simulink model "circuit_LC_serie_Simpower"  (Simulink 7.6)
settings: Solver=ode15s  StartTime=0.0  StopTime=0.0035  RelTol=1e-3
InitFcn:
  | clc, close all,clear all
  | R=10;
  | C=1e-6;
  | L=1e-3;
StopFcn:
  | close all
  | load tension_Vc.mat
  | plot(x(1,:),x(2,:))
  | hold on
  | plot(x(1,:),x(3,:))
  | %axis([0 0.04 -20 1020])
  | grid
  | title('Tension aux bornes du circuit LC série et créneau d''entrée')
  | xlabel('temps')
libraries: powerlib x9

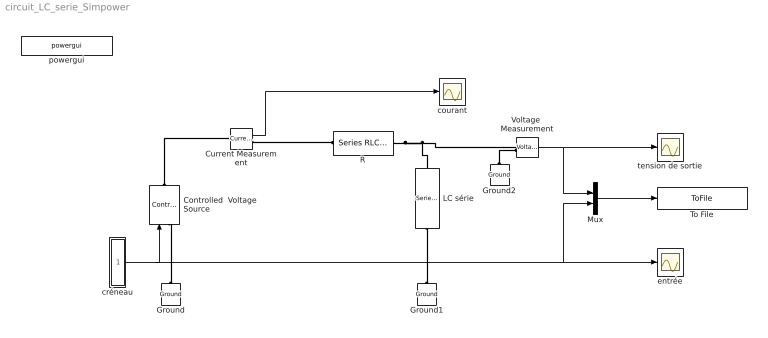
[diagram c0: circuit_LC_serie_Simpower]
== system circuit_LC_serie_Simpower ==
  Controlled  Voltage Source : powerlib/Electrical Sources/Controlled Voltage Source  DialogController=POWERSYS.PowerSysDialog  SystemSampleTime=-1  Initialize=on  Source_Type=AC  Amplitude=0  Phase=0  Frequency=0  Measurements=None
  Current Measurement : powerlib/Measurements/Current Measurement  DialogController=POWERSYS.PowerSysDialog  SystemSampleTime=-1  PhasorSimulation=off  OutputType=Complex  PSBequivalent=0
  Ground : powerlib/Elements/Ground  DialogController=POWERSYS.PowerSysDialog  PhysicalDomain=powersysdomain  SubClassName=unknown  LeftPortType=p1  RightPortType=p1  LConnTagsString=a
  Ground1 : powerlib/Elements/Ground  DialogController=POWERSYS.PowerSysDialog  PhysicalDomain=powersysdomain  SubClassName=unknown  LeftPortType=p1  RightPortType=p1  LConnTagsString=a
  Ground2 : powerlib/Elements/Ground  DialogController=POWERSYS.PowerSysDialog  PhysicalDomain=powersysdomain  SubClassName=unknown  LeftPortType=p1  RightPortType=p1  LConnTagsString=a
  LC série : powerlib/Elements/Series RLC Branch  DialogController=POWERSYS.PowerSysDialog  PhysicalDomain=powersysdomain  SubClassName=unknown  LeftPortType=p1  RightPortType=p1  LConnTagsString=__new0  RConnTagsString=__new0  BranchType=LC  Resistance=10  Inductance=L  SetiL0=off  InitialCurrent=0  Capacitance=C  Setx0=off  InitialVoltage=0  Measurements=None
  Mux : Mux  Inputs=2
  R : powerlib/Elements/Series RLC Branch  DialogController=POWERSYS.PowerSysDialog  PhysicalDomain=powersysdomain  SubClassName=unknown  LeftPortType=p1  RightPortType=p1  LConnTagsString=__new0  RConnTagsString=__new0  BranchType=R  Resistance=R  Inductance=1e-3  SetiL0=off  InitialCurrent=0  Capacitance=1e-6  Setx0=off  InitialVoltage=0  Measurements=None
  To File : ToFile  Filename=tension_Vc.mat  MatrixName=x
  Voltage  Measurement : powerlib/Measurements/Voltage Measurement  DialogController=POWERSYS.PowerSysDialog  SystemSampleTime=-1  PhasorSimulation=off  OutputType=Complex  PSBequivalent=0
  courant : Scope
  créneau : Subsystem
  entrée : Scope
  powergui : powerlib/powergui  Priority=1  SystemSampleTime=-1  SimulationMode=Continuous  SampleTime=50e-6  frequency=60  SPID=off  DisableSnubberDevices=off  DisableRonSwitches=off  DisableVfSwitches=off  SwTol=0  Interpol=off  frequencyindice=0  echomessages=off  HookPort=off  DisplayEquations=off  FunctionMessages=off  EnableUseOfTLC=off  x0status=blocks  RestoreLinks=warning  ResistiveCurrentMeasurement=off  Ylog=off  Xlog=on  ShowGrid=off  save=off  variable=ZData  ZoomFFT=off  StartTime=0.0  cycles=1  DisplayStyle=1  fundamental=60  FreqAxis=off  MaxFrequency=1000  frequencyindicesteady=1  display=off  methode=off
  tension de sortie : Scope
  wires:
  Current Measurement/1 -> courant/1
  Voltage  Measurement/1 -> tension de sortie/1, Mux/1
  créneau/1(x) -> Controlled  Voltage Source/1, entrée/1, Mux/2
  Mux/1 -> To File/1
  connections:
  Ground/LConn1 -- Controlled  Voltage Source/LConn1
  Controlled  Voltage Source/RConn1 -- Current Measurement/LConn1
  R/LConn1 -- Current Measurement/RConn1
  LC série/RConn1 -- Ground1/LConn1
  Ground2/LConn1 -- Voltage  Measurement/LConn2
  R/RConn1 -- Voltage  Measurement/LConn1 -- LC série/LConn1

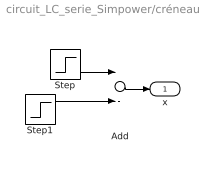
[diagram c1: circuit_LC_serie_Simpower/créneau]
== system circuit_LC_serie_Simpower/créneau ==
  Add : Sum  Inputs=+-
  Step : Step  Time=0.002  After=1000  SampleTime=0
  Step1 : Step  Time=0.0005  After=1000  SampleTime=0
  x : Outport
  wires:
  Step/1 -> Add/1
  Step1/1 -> Add/2
  Add/1 -> x/1
